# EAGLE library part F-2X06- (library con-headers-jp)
FEMALE HEADER
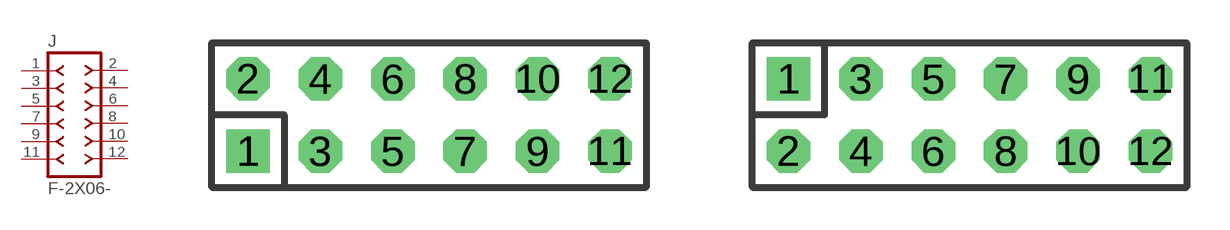
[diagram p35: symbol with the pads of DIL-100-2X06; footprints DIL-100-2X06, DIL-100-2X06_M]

Designator prefix J

## F-2X06-DIL-100  [DIL-100-2X06]
1  1  pas
2  2  pas
3  3  pas
4  4  pas
5  5  pas
6  6  pas
7  7  pas
8  8  pas
9  9  pas
10  10  pas
11  11  pas
12  12  pas

## F-2X06-DIL-100_M  [DIL-100-2X06_M]
Pads as for DIL-100-2X06

## F-2X06-DIL-2MM  [DIL-2MM-2X06]
Pads as for DIL-100-2X06

## F-2X06-DIL-2MM_M  [DIL-2MM-2X06_M]
Pads as for DIL-100-2X06

## F-2X06-71991  [71991-12]
Pads as for DIL-100-2X06

## F-2X06-79107  [79107-12]
Pads as for DIL-100-2X06

## F-2X06-79107_M  [79107-12_M]
Pads as for DIL-100-2X06

## Footprint DIL-100-2X06 (pad centres in mm)
PIN HEADER - 0.1"
drill 1.016 square: 1 -6.35,-1.27
drill 1.016 octagon: 2 -6.35,1.27; 3 -3.81,-1.27; 4 -3.81,1.27; 5 -1.27,-1.27; 6 -1.27,1.27; 7 1.27,-1.27; 8 1.27,1.27; 9 3.81,-1.27; 10 3.81,1.27; 11 6.35,-1.27; 12 6.35,1.27

## Footprint DIL-100-2X06_M (pad centres in mm)
PIN HEADER - MIRRORED 0.1"
drill 1.016 square: 1 -6.35,1.27
drill 1.016 octagon: 2 -6.35,-1.27; 3 -3.81,1.27; 4 -3.81,-1.27; 5 -1.27,1.27; 6 -1.27,-1.27; 7 1.27,1.27; 8 1.27,-1.27; 9 3.81,1.27; 10 3.81,-1.27; 11 6.35,1.27; 12 6.35,-1.27

## Footprint DIL-2MM-2X06 (pad centres in mm)
PIN HEADER - 2MM"
drill 0.711 square: 1 -5,-1
drill 0.711: 2 -5,1; 3 -3,-1; 4 -3,1; 5 -1,-1; 6 -1,1; 7 1,-1; 8 1,1; 9 3,-1; 10 3,1; 11 5,-1; 12 5,1

## Footprint DIL-2MM-2X06_M (pad centres in mm)
PIN HEADER - MIRRORED 2MM
drill 0.711 square: 1 -5,1
drill 0.711: 2 -5,-1; 3 -3,1; 4 -3,-1; 5 -1,1; 6 -1,-1; 7 1,1; 8 1,-1; 9 3,1; 10 3,-1; 11 5,1; 12 5,-1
